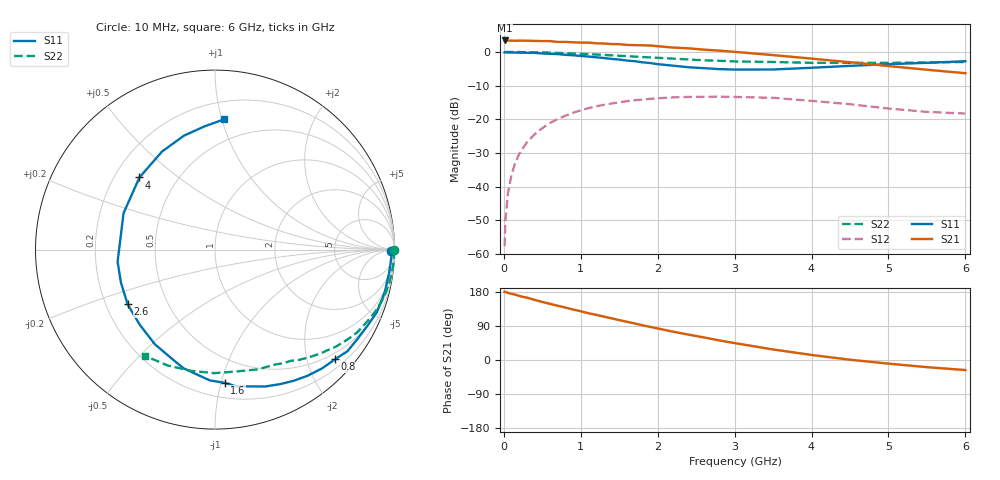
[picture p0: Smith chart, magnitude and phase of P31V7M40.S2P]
! SIEMENS Small Signal Semiconductors
! BFP181
! Si NPN RF Bipolar Junction Transistor in SOT143
! VCE = 1.75 V  IC = 0.4 mA
! Common Emitter S-Parameters:  March  1996
# GHz  S  MA  R  50
!  f  S11  S21  S12  S22
! GHz  MAG  ANG  MAG  ANG  MAG  ANG  MAG  ANG
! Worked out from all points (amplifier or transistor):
!   36 points, 10 MHz to 6 GHz, reference 50 ohm
!   highest |S21| = 3.4 dB at 10 MHz (marker M1)
!   |S21| within 3 dB of that: start of sweep to 2.786 GHz
!   unconditionally stable (mu >= 1): 3.815 GHz to end of sweep
!   at 250 MHz: K = 0.08, MSG = 15.9 dB, |S12| = -28.5 dB
!   at 1.4 GHz: K = 0.44, MSG = 8.8 dB, |S12| = -15.3 dB
!   at 6 GHz: K = 1.51, MAG = 1.8 dB, |S12| = -18.3 dB
!   S11 on the Smith chart (normalised r, x): 10 MHz: 84, -49; 800 MHz: 0.37, -2.53; 1.6 GHz: 0.31, -1.03; 2.6 GHz: 0.29, -0.27; 4 GHz: 0.30, +0.37; 6 GHz: 0.33, +1.02
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0.01  0.9824 -0.6  1.481 179.9  0.0013 90.0  0.9994 -0.2
0.02  0.9886 -0.9  1.478 179.7  0.0031 84.9  0.999 -0.5
0.05  0.9833 -2.4  1.475 177.4  0.0076 91.0  0.9985 -1.4
0.1  0.9804 -5.2  1.47 174.8  0.015 83.5  0.9978 -2.7
0.15  0.9786 -7.9  1.463 172.2  0.0228 83.6  0.9968 -3.9
0.2  0.9751 -10.8  1.472 169.3  0.0304 82.0  0.9964 -5.3
0.3  0.9716 -16.0  1.466 164.6  0.0453 78.3  0.993 -8.0
0.4  0.9667 -21.2  1.458 158.6  0.0597 74.4  0.989 -10.6
0.6  0.9372 -32.0  1.449 148.3  0.0878 66.5  0.9766 -15.8
0.8  0.9058 -42.4  1.409 138.3  0.1128 59.0  0.9589 -20.7
1.1  0.8528 -58.9  1.374 123.5  0.146 48.3  0.9268 -27.7
1.5  0.7703 -81.3  1.304 105.3  0.1783 35.1  0.8763 -36.4
1.6  0.7441 -85.9  1.273 100.8  0.1855 32.3  0.8674 -38.2
1.9  0.6842 -104.8  1.246 87.5  0.201 23.3  0.8278 -44.0
2.2  0.6249 -122.4  1.161 74.7  0.2111 15.4  0.7955 -49.1
2.6  0.5743 -147.9  1.081 59.6  0.2153 5.9  0.7504 -55.6
3  0.5469 -172.9  1.003 44.6  0.2145 -3.6  0.7231 -62.2
3.5  0.5485 158.3  0.897 27.8  0.208 -13.0  0.7087 -70.3
4  0.582 136.3  0.796 13.3  0.1874 -20.5  0.6896 -79.9
4.5  0.6209 118.4  0.703 0.7  0.1671 -26.2  0.6885 -90.4
5.5  0.6893 94.8  0.544 -18.9  0.1287 -25.0  0.6974 -112.3
6  0.7275 86.0  0.483 -26.5  0.1214 -20.1  0.7093 -123.6
